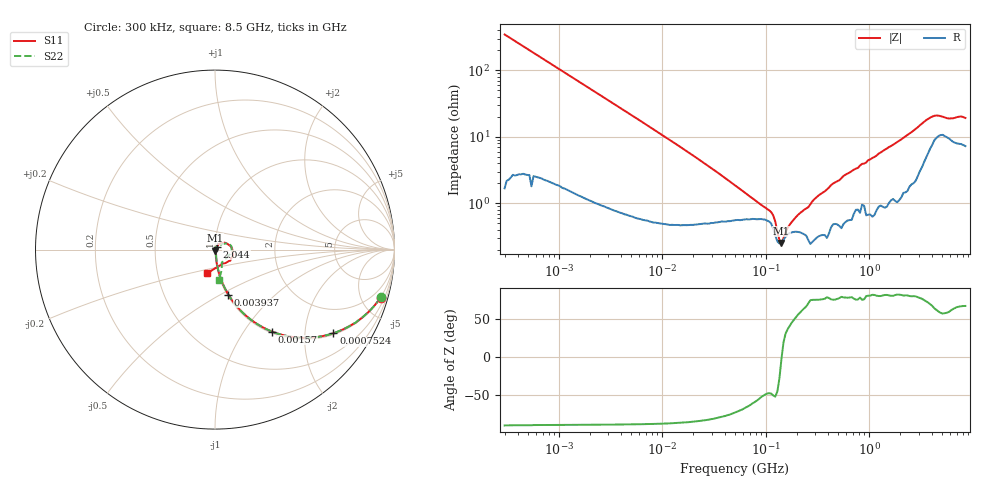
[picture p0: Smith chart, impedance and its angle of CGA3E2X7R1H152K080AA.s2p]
! S-parameter Generated by TDK Corporation
! Copyright(C) 2015 TDK Corporation.
! All Rights Reserved.
! TDK P/N: CGA3E2X7R1H152K080AA (Multilayer Ceramic Chip Capacitors)
! Property: C=1.5nF
! Size(LxWxT): 1.6x0.8x0.8mm, 0.063x0.031x0.031inches
! Model Type: s2p (Touchstone File Format Version 1.0)
! Frequency: DC=Yes Start=0.3MHz Stop=8500MHz 225points Log-sweep
! Note:
! Model Generated on Jun. 23, 2015
! Hash(MD5):
! Port Assignments:
!  1 ---| |--- 2
! Applicable Conditions:
!  Temperature = 25 degC
!  DC Bias Voltage = 0 V
!  Small Signal Operation
! Terms and conditions regarding TDK Simulation Models
! (1)This simulation model is being provided solely for informational purposes. Please refer to the specifications of the products in terms of detailed characteristics of such products.
! (2)In no event shall TDK Corporation of any of its subsidiaries be liable for any loss or damage arising, directly or indirectly,
!  From any information contained in this simulation model, including, but not limited to loss or damages arising from any inaccuracies, omissions or errors in connection with such information.
! (3)Any and all copyrights on this simulation model are owned by TDK Corporation.
!  Duplication or redistribution of this simulation model without prior written permission from TDK Corporation is prohibited.
! (4)This simulation model is subject to any modification or change without any prior notice.
! (5)Neither TDK Corporation nor any of its subsidiaries shall make any warranty, express or implied,
!  Including but not limited to the correctness, implied warranties of merchantability and fitness for a particular purpose with respect to this simulation models.
! (6)The use of this simulation model shall be deemed to have consented to the terms and conditions hereof.
# MHz S MA R 50
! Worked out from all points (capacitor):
!   224 points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, 300 kHz to 8.5 GHz, reference 50 ohm
!   read as one part in series: C = 1.52 nF near 314.1 kHz
!   lowest |Z| = 252 mohm at 142.1 MHz (marker M1)
!   series resonance near 142.5 MHz, so ESL is about 820 pH
!   S11 on the Smith chart (normalised r, x): 300 kHz: 1.01, -6.90; 752.4 kHz: 1.05, -2.80; 1.57 MHz: 1.02, -1.35; 3.937 MHz: 1.01, -0.54; 2.044 GHz: 1.02, +0.03; 8.5 GHz: 0.88, -0.24
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0.3  0.9602 -16.2  0.2769 73.6  0.277 73.9  0.9603 -16.1
0.7523683  0.8073 -35.3  0.5773 53.9  0.5761 54.1  0.8073 -35.3
1.569921  0.5559 -55.2  0.8223 33.7  0.8207 33.9  0.5558 -55.2
1.72111  0.5215 -57.5  0.8447 31.3  0.8432 31.5  0.5213 -57.5
3.937196  0.2611 -73.5  0.9597 15.0  0.9582 15.2  0.2608 -73.5
9.430415  0.1126 -81.3  0.9895 6.3  0.9881 6.5  0.1124 -81.2
51.67171  0.01873 -76.9  0.9944 0.8  0.9933 1.0  0.02153 -72.1
142.0669  0.005088 -84.5  0.9972 -0.4  0.9958 -0.2  0.006499 -66.2
195.9978  0.001065 -153.6  0.9944 -0.9  0.993 -0.6  0.006786 -61.2
246.6485  0.00155 153.7  0.9934 -1.1  0.9922 -0.9  0.004792 -90.4
283.1228  0.002663 -171.2  0.9941 -1.4  0.9928 -1.1  0.001226 -82.3
310.3886  0.002449 -177.3  0.9932 -1.5  0.992 -1.3  0.0003904 -116.4
390.6008  0.0007838 -134.7  0.9932 -1.9  0.992 -1.6  0.003751 123.5
590.7752  0.00319 74.2  0.9907 -2.9  0.9897 -2.6  0.006451 79.0
678.1388  0.002035 65.2  0.9902 -3.3  0.9892 -3.0  0.009394 78.5
893.5346  0.01314 45.5  0.9893 -4.1  0.9885 -3.9  0.007547 32.6
1124.446  0.006817 73.1  0.9891 -5.4  0.9878 -5.1  0.008861 66.3
1551.304  0.01452 58.0  0.9856 -7.3  0.9846 -7.0  0.0167 64.7
2044.041  0.01923 57.9  0.9836 -9.6  0.9822 -9.2  0.0204 55.3
4265.177  0.08999 11.3  0.9114 -18.8  0.9108 -18.5  0.09365 11.1
6450.987  0.09674 -46.6  0.9126 -23.2  0.9102 -22.8  0.08081 -60.4
8500  0.1407 -109.1  0.9045 -31.0  0.9041 -30.2  0.1727 -83.0
